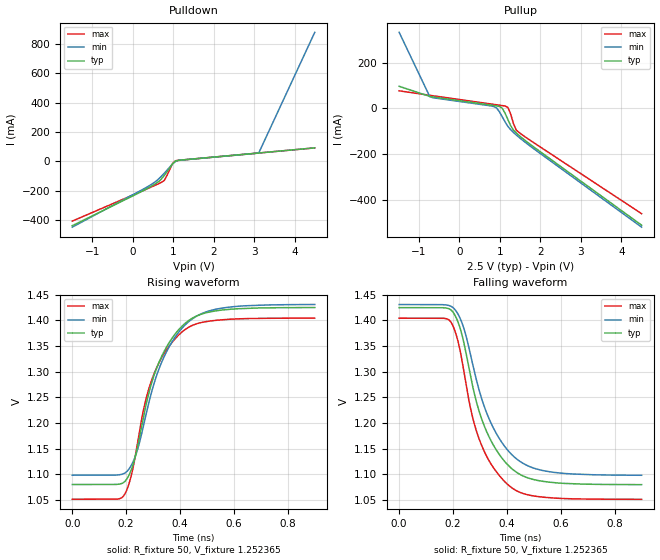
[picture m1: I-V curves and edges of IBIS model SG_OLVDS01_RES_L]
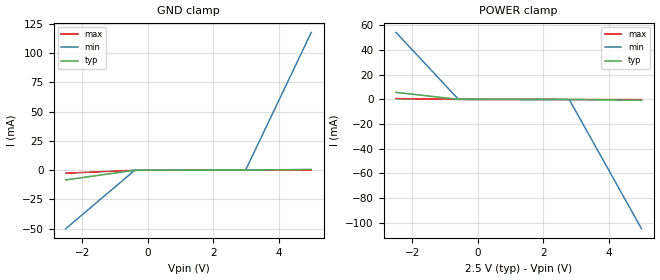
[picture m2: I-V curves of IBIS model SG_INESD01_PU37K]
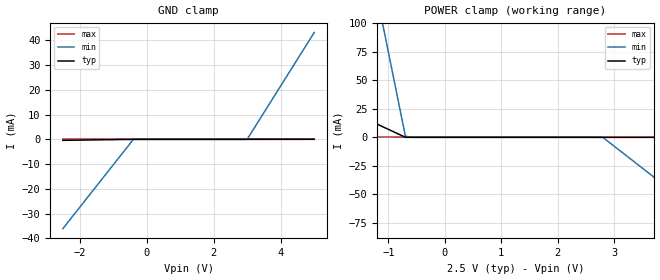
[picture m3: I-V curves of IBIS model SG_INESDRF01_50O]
|   This file is an IBIS representation of the   |
|   Integrated Device Technology Inc   |
|   ICS8S89832I   |
|   LOW SKEW, 1-TO-4 DIFFERENTIAL-TO-LVDS FANOUT BUFFER   |
[IBIS Ver]   4.1
[File name]   8s89832i_2v5.ibs
[File Rev]   1.0
[Date]   9 Feb 2010
[Source]   Originated at Integrated Device Technology, Inc.
[Disclaimer]
IDT hereby grants the user of this IBIS model a non-exclusive,
nontransferable license to use this IBIS model under the following terms.
Before using this IBIS model, the user should read this license.
If the user does not accept these terms,  the IBIS model should be
returned to IDT within 30 days.
   The user is granted this license only to use the IBIS model and
is not granted rights to sell, load, rent, lease or license the IBIS
model in whole or in part, or in modified form to anyone other than
user. User may modify the IBIS model to suit its specific
applications but rights to derivative works and such modifications
shall belong to IDT.
   This IBIS model is provided on an "AS IS" basis and IDT makes
absolutely no warranty with respect to the information contained
herein. IDT DISCLAIMS AND CUSTOMER WAIVES ALL WARRANTIES, EXPRESS
OR IMPLIED, INCLUDING WARRANTIES OF MERCHANTABILITY OR FITNESS FOR
A PARTICULAR PURPOSE. The entire risk as to quality and performance
is with the Customer. ACCORDINGLY, IN NO EVENT SHALL THE COMPANY BE
LIABLE FOR ANY DAMAGES, WHETHER IN CONTRACT OR TORT,INCLUDING ANY
LOST PROFITS OR OTHER INCIDENTAL, CONSEQUENTIAL, EXEMPLARY, OR
PUNITIVE DAMAGES ARISING OUT OF THE USE OR APPLICATION OF THE IBIS
model provided in this package. Further, IDT reserves the right to
make changes without notice to any product herein to improve
reliability, function, or design. IDT does not convey any license
under patent rights or any other intellectual property rights,
including those of third parties.
   IDT is not obligated to provide maintenance or support
for the licensed IBIS model.
[Copyright]   Copyright 2010 by IDT Inc.
[Component]   ICS8S89832KI
[Manufacturer] Integrated Device Technology, Inc.
[Package]
|QFN 16
|lead + wire   typ   min   max
R_pkg   72.4655m   58.886m   86.045m
L_pkg   1.47175nH   1.11650nH   1.77850n
C_pkg   0.07747pF   0.07444pF   0.08050pF
[Pin] signal_name  model_name   R_pin   L_pin   C_pin
1   Q1   SG_OLVDS01_RES_L   86.045m   1.77850nH   0.08050pF
2   nQ1   SG_OLVDS01_RES_L   58.886m   1.11650nH   0.07444pF
3   Q2   SG_OLVDS01_RES_L   58.886m   1.11650nH   0.07444pF
4   nQ2   SG_OLVDS01_RES_L   86.045m   1.77850nH   0.08050pF
5   Q3   SG_OLVDS01_RES_L   86.045m   1.77850nH   0.08050pF
6   nQ3   SG_OLVDS01_RES_L   58.886m   1.11650nH   0.07444pF
7   VDD   POWER   58.886m   1.11650nH   0.07444pF
8   EN   SG_INESD01_PU37K   86.045m   1.77850nH   0.08050pF
9   nIN   SG_INESDRF01_50O   86.045m   1.77850nH   0.08050pF
10   VREF_AC  NC   58.886m   1.11650nH   0.07444pF
11   VT   SG_VTERM02   58.886m   1.11650nH   0.07444pF
12   IN   SG_INESDRF01_50O   86.045m   1.77850nH   0.08050pF
13   GND   GND   86.045m   1.77850nH   0.08050pF
14   VDD   POWER   58.886m   1.11650nH   0.07444pF
15   Q0   SG_OLVDS01_RES_L   58.886m   1.11650nH   0.07444pF
16   nQ0   SG_OLVDS01_RES_L   86.045m   1.77850nH   0.08050pF
[Diff Pin]  inv_pin   vdiff   tdelay_typ   tdelay_min   tdelay_max
|Output
1   2   NA   0   0   0
3   4   NA   0   0   0
5   6   NA   0   0   0
15   16   NA   0   0   0
|Input
12   9   0.3   0   0   0
[Series Pin Mapping] Pin_2   model_name   function_table_group
12   9   ODT_100
[Model]   ODT_100
Model_type  Series
Polarity   Non-Inverting
|   typ   min   max
C_comp   0pF   0pF   0pF
|   typ   min   max
[Voltage Range]   2.5V   2.375V   2.625V
[R Series]   100ohm   100ohm   100ohm
| Models and submodels in the file (5): ODT_100 (Series), SG_OLVDS01_RES_L (Output), SG_INESD01_PU37K (Input), SG_INESDRF01_50O (Input), SG_VTERM02 (Input)
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[Model]   SG_OLVDS01_RES_L
Model_type   Output
Polarity   Non-Inverting
|   typ   min   max
C_comp   2pF   1.5pF   2.5pF
Vmeas = 1.252V
Rref = 50
Cref = 0
Vref = 1.252V
|   typ   min   max
[Voltage range]   2.5V   2.375V   2.625V
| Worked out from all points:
|   slope of the pulldown table from 0 to 0.375 V, typ, clamps not added: 7.04 ohm
|   slope of the pullup table from 0 to 0.375 V, typ, clamps not added: 40 ohm
|   rising waveform, R_fixture 50, V_fixture 1.252365: 20-80 % time 118ps typ, 127ps min, 110ps max; typ from 1.08 V to 1.43 V
|   falling waveform, R_fixture 50, V_fixture 1.252365: 20-80 % time 118ps typ, 127ps min, 110ps max; typ from 1.43 V to 1.08 V
[Pulldown]
|Voltage   I (typ)   I (min)   I (max)
-1.49V    -438.6mA   -448.5mA   -407.2mA
300.1mV   -194mA     -183.6mA   -194.3mA
575.5mV   -150.8mA   -135.8mA   -160.6mA
713.2mV   -119.4mA   -100.8mA   -142.5mA
782.1mV   -95.79mA   -81mA      -130.4mA
988.6mV   -16.25mA   -16.49mA   -14.12mA
1.057V    1.823mA    -420.3uA   4.178mA
1.195V    9.23mA     8.619mA    9.027mA
2.985V    53.96mA    53.22mA    54.03mA
3.123V    57.4mA     61.3mA     57.49mA
4.5V      92.44mA    880.4mA    92.11mA
[Pullup]
|Voltage   I (typ)   I (min)   I (max)
-1.49V    96.84mA    332.8mA    76.94mA
-732.6mV  52.4mA     51.41mA    57.32mA
850.9mV   12.68mA    8.278mA    17.51mA
919.8mV   10.91mA    1.327mA    15.78mA
988.6mV   8.546mA    -15.16mA   14.05mA
1.057V    686.3uA    -36.83mA   12.31mA
1.195V    -48.35mA   -78.3mA    4.556mA
1.264V    -75.08mA   -92.72mA   -23.98mA
1.333V    -94.5mA    -104.8mA   -65.89mA
1.402V    -107.1mA   -115.8mA   -94.6mA
1.539V    -128.4mA   -136.2mA   -114mA
4.5V      -510.8mA   -519.3mA   -460.3mA
[Ramp]
|   typ   min   max
dV/dt_r   0.276/0.188n   0.266/0.201n   0.282/0.177n
dV/dt_f   0.276/0.188n   0.266/0.201n   0.282/0.177n
R_load =   50.0000
[Rising Waveform]
R_fixture = 50
V_fixture   =1.252365   |Vcc_typ
V_fixture_min=1.264475  |Vcc_min
V_fixture_max=1.227695  |Vcc_max
C_fixture = 0.0p
| Time   typ   min   max
0s        1.08V      1.098V     1.051V
192.8ps   1.085V     1.101V     1.059V
216.2ps   1.105V     1.115V     1.092V
237.8ps   1.143V     1.141V     1.147V
266.7ps   1.218V     1.2V       1.231V
297.3ps   1.283V     1.266V     1.287V
349.5ps   1.348V     1.339V     1.342V
416.2ps   1.393V     1.39V      1.381V
554.1ps   1.42V      1.424V     1.401V
900ps     1.425V     1.431V     1.405V
[Falling Waveform]
R_fixture = 50
V_fixture   =1.252365   |Vcc_typ
V_fixture_min=1.264475  |Vcc_min
V_fixture_max=1.227695  |Vcc_max
C_fixture = 0.0p
| Time   typ   min   max
0s        1.425V     1.431V     1.404V
192.8ps   1.42V      1.428V     1.396V
216.2ps   1.4V       1.414V     1.364V
237.8ps   1.362V     1.388V     1.308V
266.7ps   1.287V     1.329V     1.224V
297.3ps   1.222V     1.263V     1.168V
349.5ps   1.157V     1.19V      1.113V
416.2ps   1.112V     1.139V     1.074V
554.1ps   1.085V     1.105V     1.054V
900ps     1.08V      1.098V     1.051V
[Model]   SG_INESD01_PU37K
Model_type   Input
Polarity   Non-Inverting
Vinl = 0.8V
Vinh = 2.2V
|   typ   min   max
C_comp   2pF   1.5pF   2.5pF
|   typ   min   max
[Voltage range]   2.5V   2.375V   2.625V
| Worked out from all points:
|   GND clamp passes 1 mA (typ) near -0.63 V on its own axis
|   POWER clamp passes 1 mA (typ) near -0.92 V on its own axis
[GND_clamp]
|Voltage   I (typ)   I (min)   I (max)
-2.5V     -8.291mA   -49.95mA   -2.608mA
-400mV    -106.4uA   -232.7uA   -107.9uA
3V        15.41uA    485.5uA    13uA
5V        659uA      117.7mA    82.51uA
[Power_clamp]
|Voltage   I (typ)   I (min)   I (max)
-2.5V     5.693mA    54.38mA    628.9uA
-600mV    47.59uA    280.9uA    22.09uA
2.8V      -75.28uA   -402.4uA   -97.1uA
5V        -760.2uA   -104.9mA   -173.7uA
[Model]   SG_INESDRF01_50O
Model_type   Input
Polarity   Non-Inverting
Vinl = 0.8V
Vinh = 2.2V
|   typ   min   max
C_comp   2pF   1.5pF   2.5pF
|   typ   min   max
[Voltage range]   2.5V   2.375V   2.625V
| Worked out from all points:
|   POWER clamp passes 1 mA (typ) near -0.74 V on its own axis
[GND_clamp]
|Voltage   I (typ)   I (min)   I (max)
-2.5V     -396.9uA   -36.05mA   -256.7nA
-400mV    -393.2nA   -69.82uA   -92.43pA
3V        19.97nA    87.82uA    12.78pA
5V        19.18uA    43.19mA    118.6pA
[Power_clamp]
|Voltage   I (typ)   I (min)   I (max)
-2.5V     41.5mA     441.7mA    895.4uA
-1.1V     9.259mA    98.93mA    199.2uA
-1V       6.956mA    74.44mA    149.5uA
-700mV    47.95uA    997.7uA    345.1nA
-500mV    19.97nA    1.53uA     29.89pA
2.8V      -8.026nA   -157uA     -6.301pA
5V        -8.481uA   -84.9mA    -23.18pA
